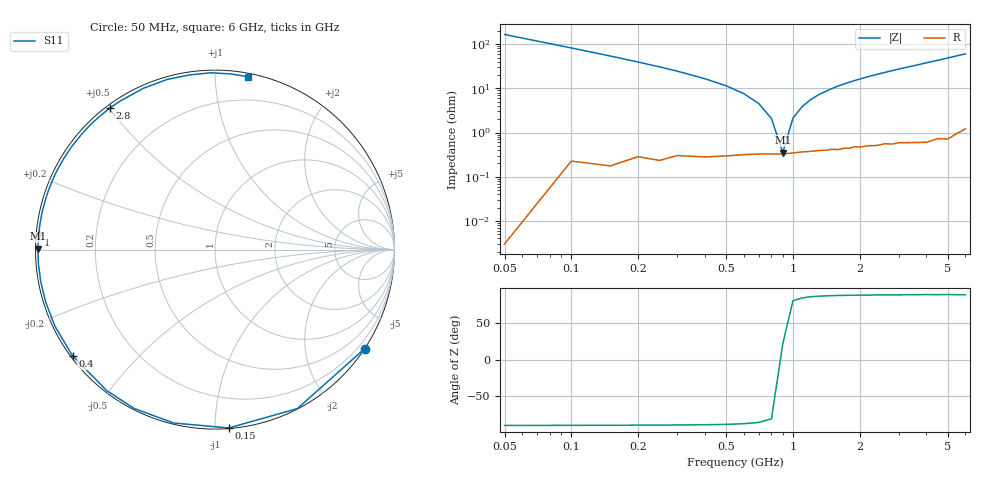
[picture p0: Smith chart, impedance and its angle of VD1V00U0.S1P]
! Infineon Technologies  Discrete & RF Semiconductors
! BBY 55-03
! Si Tuning Diode in SOD323
! VR = 1 V
! S-Parameters:  June  1999
# GHz  S  MA  R  50
!  f  S11
! GHz  MAG  ANG
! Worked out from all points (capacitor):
!   34 points, 50 MHz to 6 GHz, reference 50 ohm
!   read as one part to ground: C = 19.1 pF near 50 MHz
!   lowest |Z| = 353 mohm at 900 MHz (marker M1)
!   series resonance near 894 MHz, so ESL is about 1.7 nH
!   S11 on the Smith chart (normalised r, x): 50 MHz: 0.00, -3.32; 150 MHz: 0.00, -1.08; 400 MHz: 0.01, -0.33; 1 GHz: 0.01, +0.04; 2.8 GHz: 0.01, +0.50; 6 GHz: 0.02, +1.21
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0.05  1 -33.5
0.1  0.9976 -62.6
0.15  0.9968 -85.6
0.2  0.993 -103.4
0.25  0.9932 -116.9
0.3  0.9903 -127.6
0.4  0.9899 -143.3
0.5  0.9888 -154.3
0.6  0.9877 -162.7
0.7  0.9872 -169.6
0.8  0.987 -175.3
0.9  0.987 179.7
1  0.9863 175.2
1.2  0.9853 167.4
1.3  0.9848 163.9
1.6  0.9845 154.6
1.8  0.9837 149.1
2  0.9831 144.0
2.2  0.9824 139.2
2.4  0.9828 134.8
2.8  0.9826 126.6
3  0.9821 122.7
3.5  0.9834 114.0
4  0.9849 105.7
4.5  0.9835 98.2
5  0.9855 91.4
5.5  0.9827 84.9
6  0.9805 79.2
